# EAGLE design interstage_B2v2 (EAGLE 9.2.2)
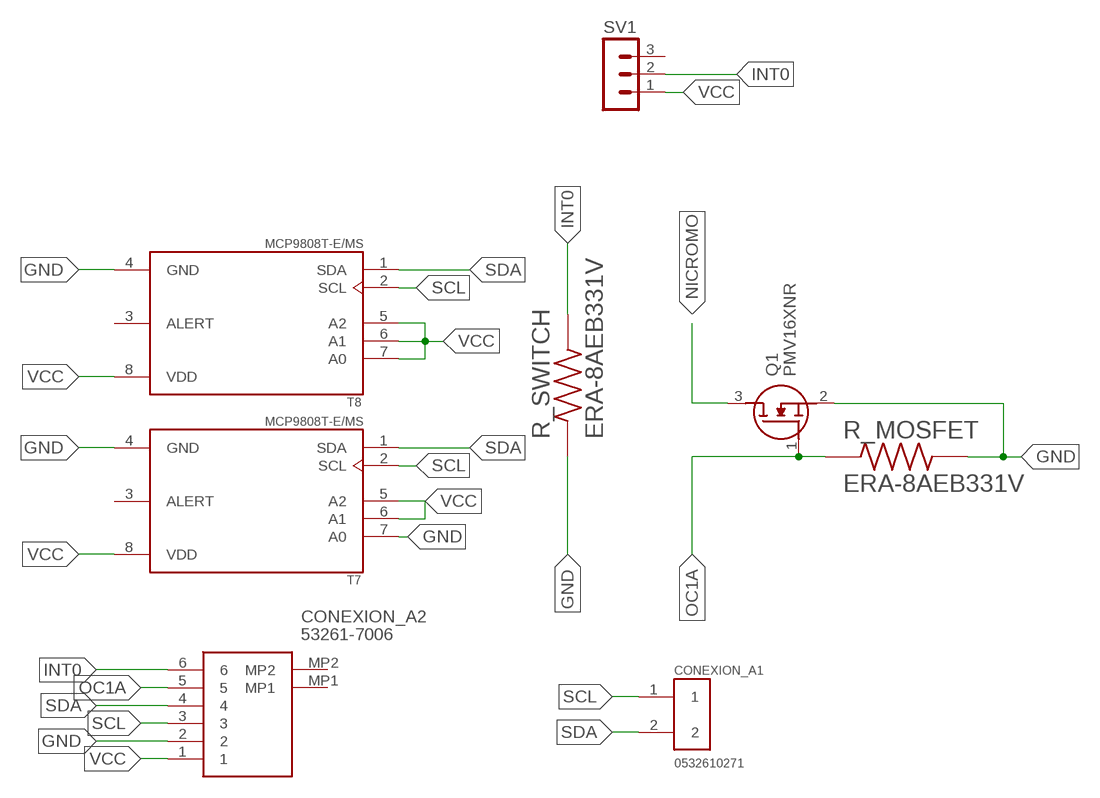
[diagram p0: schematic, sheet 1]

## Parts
CONEXION_A1  0532610271  [MOLEX_0532610271]
CONEXION_A2  53261-7006  [532617006]
Q1  PMV16XNR  [SOT95P230X110-3N]
R_MOSFET  ERA-8AEB331V  [RESC3216X70N]
R_SWITCH  ERA-8AEB331V  [RESC3216X70N]
SV1  MA03-1  [MA03-1]
T7  MCP9808T-E/MS  [SOP65P490X110-8N]
T8  MCP9808T-E/MS  [SOP65P490X110-8N]

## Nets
GND: CONEXION_A2.2 Q1.2(S) R_MOSFET.2 R_SWITCH.1 T7.4(GND) T7.7(A0) T8.4(GND)
INT0: CONEXION_A2.6 R_SWITCH.2 SV1.2
NICROMO: Q1.3(D)
OC1A: CONEXION_A2.5 Q1.1(G) R_MOSFET.1
SCL: CONEXION_A1.1 CONEXION_A2.3 T7.2(SCL) T8.2(SCL)
SDA: CONEXION_A1.2 CONEXION_A2.4 T7.1(SDA) T8.1(SDA)
VCC: CONEXION_A2.1 SV1.1 T7.5(A2) T7.6(A1) T7.8(VDD) T8.5(A2) T8.6(A1) T8.7(A0) T8.8(VDD)
Unconnected: CONEXION_A2.MP1 CONEXION_A2.MP2 SV1.3 T7.3(ALERT) T8.3(ALERT)

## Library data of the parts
CONEXION_A1 = picoblade2:0532610271: 1.25mm (.049") Pitch PicoBlade Header, Surface Mount, Right Angle, Lead-free, 2 Circuits; AVAILABILITY: Unavailable; DESCRIPTION: Picoblade Connector, 2 Circuit Single Row, Right Angle Surface Mount SMT PCB; DIGIKEY-PURCHASE-URL: https://snapeda.com/shop?store=DigiKey&id=4477935; MF: Molex; MP: 0532610271; PACKAGE: None; PRICE: None
CONEXION_A2 = SamacSys_Parts:53261-7006: 1.25mm Pitch, PicoBlade PCB Header, Single Row, Right-Angle, Surface Mount, Gold (Au) Plating, Friction Lock, Circuits, Tape and Reel Source: Datasheet; DESCRIPTION: 1.25mm Pitch, PicoBlade PCB Header, Single Row, Right-Angle, Surface Mount, Gold (Au) Plating, Friction Lock, Circuits, Tape and Reel; HEIGHT: 3.6mm; MANUFACTURER_NAME: Molex; MANUFACTURER_PART_NUMBER: 53261-7006; MOUSER_PART_NUMBER: 538-53261-7006; MOUSER_PRICE-STOCK: https://www.mouser.co.uk/ProductDetail/Molex/53261-7006?qs=0lSvoLzn4L%2FSBef0BTU2GA%3D%3D
Q1 = SamacSys_Parts:PMV16XNR: Nexperia PMV16XNR N-channel MOSFET, 8.6 A, 20 V PMV16XN, 3-Pin SOT-23 Source: Datasheet; DESCRIPTION: Nexperia PMV16XNR N-channel MOSFET, 8.6 A, 20 V PMV16XN, 3-Pin SOT-23; HEIGHT: 1.1mm; MANUFACTURER_NAME: Nexperia; MANUFACTURER_PART_NUMBER: PMV16XNR; MOUSER_PART_NUMBER: 771-PMV16XNR; MOUSER_PRICE-STOCK: https://www.mouser.com/Search/Refine.aspx?Keyword=771-PMV16XNR
R_MOSFET R_SWITCH = resistor_330_smd:ERA-8AEB331V; DESCRIPTION: 330 Ohms ±0.1% 0.25W, 1/4W Chip Resistor 1206 (3216 Metric) Automotive AEC-Q200 Thin Film; DIGI-KEY_PART_NUMBER: P330BCCT-ND; MF: Panasonic Electronic; MP: ERA-8AEB331V; PACKAGE: 3216 Panasonic Electronic Components
SV1 = con-lstb:MA03-1: PIN HEADER; OC_FARNELL: unknown; OC_NEWARK: unknown
T7 T8 = sensorSPEL:MCP9808T-E/MS: Board Mount Temperature Sensors Silicon temp sensor with I2C interface; DESCRIPTION: Temperature Sensor Digital, Local -40°C ~ 125°C 10 b 8-MSOP; DIGI-KEY_PART_NUMBER: MCP9808T-E/MSCT-ND; MF: Microchip; MP: MCP9808T-E/MS; PACKAGE: MSOP-8 Microchip

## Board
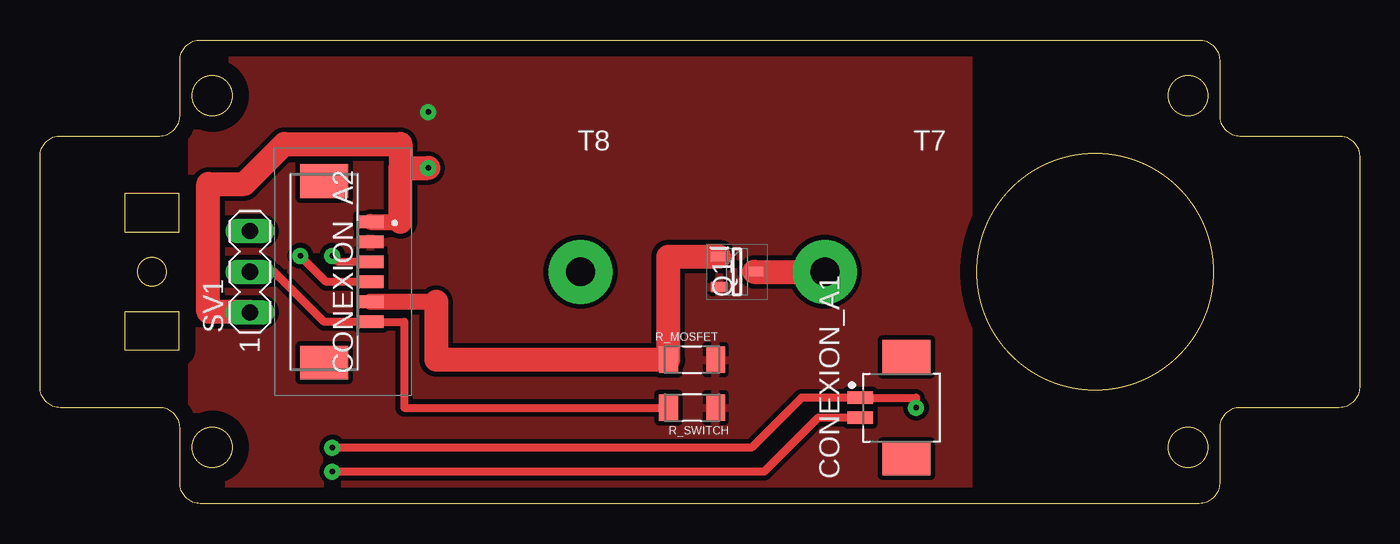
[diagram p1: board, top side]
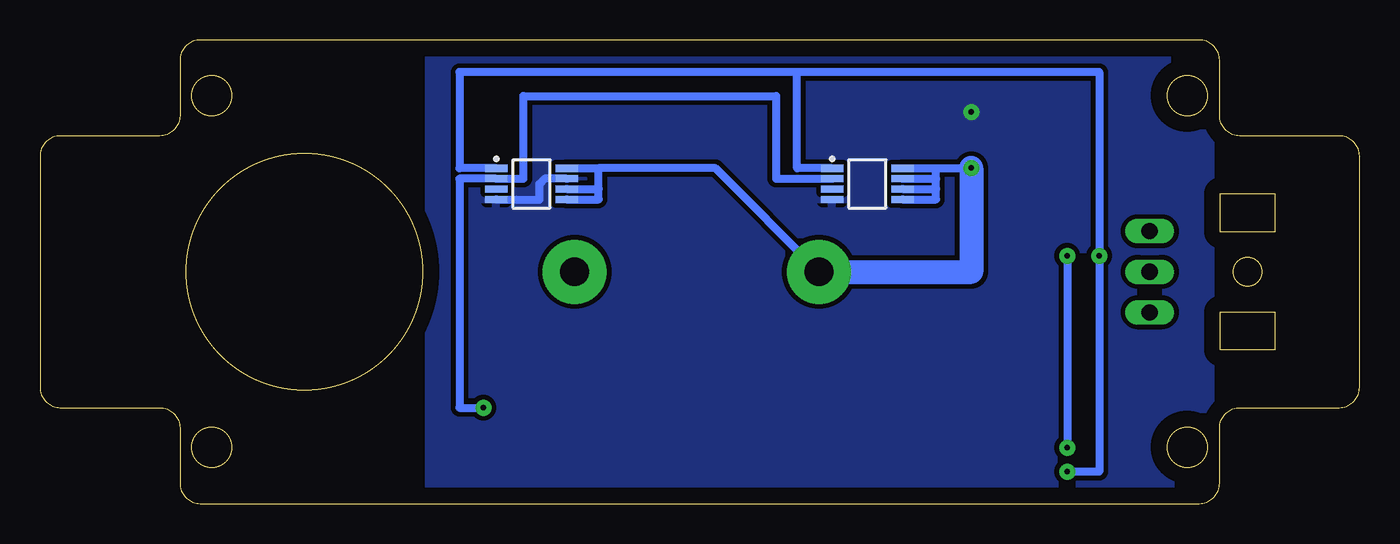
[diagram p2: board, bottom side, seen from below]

Size 82.5 x 29 mm. Coordinates in mm from the lower left corner, seen from the top.
Outline: 8.7,17 8.7,19.4 5.3,19.4 5.3,17 8.7,17
Outline: 8.7,9.6 8.7,12 5.3,12 5.3,9.6 8.7,9.6
Outline: 82.5,21.73 82.5,7.27 arc-90 81.23,6 75.02,6 arc90 73.75,4.73 73.75,1.27 arc-90 72.48,0 10.02,0 arc-90 8.75,1.27 8.75,4.73 arc90 7.48,6 1.27,6 arc-90 0,7.27 0,21.73 arc-90 1.27,23 7.48,23 arc90 8.75,24.27 8.75,27.73 arc-90 10.02,29 72.48,29 arc-90 73.75,27.73 73.75,24.27 arc90 75.02,23 81.23,23 arc-90 82.5,21.73
Outline: circle at 7,14.5 radius 0.9
Outline: circle at 65.97,14.5 radius 7.4
Outline: circle at 71.78,3.52 radius 1.25
Outline: circle at 10.77,25.52 radius 1.25
Outline: circle at 10.77,3.52 radius 1.25
Outline: circle at 71.78,25.52 radius 1.25
Copper layers (1*16): Top 0.035mm / dielectric 1.5mm / Bottom 0.035mm
Design rules "default *": minimum track width 6mil, minimum drill 0.35mm, track to track 0.3mm, track to pad 6mil, pad to pad 6mil, via to via 6mil, smd to smd 6mil, copper to edge 40mil, drill to drill 6mil, minimum pad ring 10mil, minimum via ring 8mil, stop-mask expansion 4mil, vias tented up to drill 0mil, thermal gap 10mil

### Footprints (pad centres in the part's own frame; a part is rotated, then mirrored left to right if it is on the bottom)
MOLEX_0532610271 = smd 0.8 x 1.6: 1 0.625,0; 2 -0.625,0 | smd 2.1 x 3: 3 -3.175,-2.9; 4 3.175,-2.9
532617006 = smd 0.8 x 1.6: 1 3.125,-2.5; 2 1.875,-2.5; 3 0.625,-2.5; 4 -0.625,-2.5; 5 -1.875,-2.5; 6 -3.125,-2.5 | smd 2.1 x 3: MP1 5.675,0.4; MP2 -5.675,0.4
SOT95P230X110-3N = smd 1.05 x 0.6: 1 -1.1,0.95; 2 -1.1,-0.95; 3 1.1,0
RESC3216X70N = smd 1.16 x 1.68: 1 -1.475,0; 2 1.475,0
MA03-1 = drill 1.016 long: 1 -2.54,0; 2 0,0; 3 2.54,0
SOP65P490X110-8N = smd 1.4 x 0.45: 1 -2.2,0.975; 2 -2.2,0.325; 3 -2.2,-0.325; 4 -2.2,-0.975; 5 2.2,-0.975; 6 2.2,-0.325; 7 2.2,0.325; 8 2.2,0.975

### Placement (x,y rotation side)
CONEXION_A1  51.27,6 90 top
CONEXION_A2  18.17,14.5 90 top
Q1  43.57,14.5 0 top
R_MOSFET  40.77,9 0 top
R_SWITCH  40.77,6 180 top
SV1  13.12,14.5 90 top
T7  51.77,20 0 bottom
T8  30.77,20 0 bottom

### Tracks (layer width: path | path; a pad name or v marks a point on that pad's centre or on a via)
GND  (via drill 0.35 pad 1)
  Bottom 0.5: T7.7 50.94,20.32 51.27,20 51.27,19 51.3,19.02 T7.4
  other vias: 24.27,24.5
  pour Top: 9.47,28 9.47,0.6 58.07,0.6 58.07,28.1 57.97,28
  pour Bottom: 9.32,28 9.32,0.4 58.17,0.4 58.17,28
INT0
  Top 0.5: SV1.2 14.64,14.5 17.77,11.38 CONEXION_A2.6 22.77,11.38 22.77,6 R_SWITCH.2
NICROMO  (via drill 1.8 pad 4)
  Top 1.5: Q1.3 v49.07,14.5
OC1A
  Top 0.5: R_MOSFET.1 39.27,9.03
  Top 1: 24.77,12.62 CONEXION_A2.5
  Top 1.5: Q1.1 39.27,15.45 39.27,9.03 | 24.77,12.62 24.77,9 R_MOSFET.1
SCL  (via drill 0.35 pad 1)
  Top 0.5: v54.77,6 54.77,6.62 CONEXION_A1.1 47.59,6.62 44.47,3.5 v18.27,3.5 | CONEXION_A2.3 18.64,15.12 v18.27,15.5
  Bottom 0.5: T8.2 36.47,20.32 36.47,25.5 52.27,25.5 52.27,20.32 T7.2 56.27,20.32 56.27,6 v54.77,6 | v18.27,15.5 v18.27,3.5
SDA  (via drill 0.35 pad 1)
  Top 0.5: CONEXION_A1.2 48.64,5.38 45.27,2 v18.27,2 | CONEXION_A2.4 17.89,13.88 v16.27,15.5
  Bottom 0.5: T8.1 35.17,20.98 35.17,27 | T7.1 56.27,20.98 56.27,27 35.17,27 | 35.17,27 16.27,27 v16.27,15.5 16.27,2 v18.27,2
VCC  (via drill 0.35 pad 1, 1.8 pad 4)
  Top 0.5: SV1.1 13.08,12
  Top 1: CONEXION_A2.1 22.55,17.62
  Top 1.5: 22.55,17.62 22.55,21 | 22.55,21 v24.27,21 | 13.08,12 10.52,12 10.52,20 12.77,20 15.27,22.5 22.55,22.5 22.55,21
  Bottom 0.5: T8.8 26.47,20.98 | T7.8 47.57,20.98 | T8.7 26.47,20.32 | 26.47,20.32 26.47,20.98 | T8.6 26.47,19.68 | 26.47,19.68 26.47,20.32 | T8.5 26.47,19.02 26.47,19.68 | T7.6 47.57,19.68 | 47.57,19.68 47.57,20.98 | T7.5 47.57,19.02 47.57,19.68 | 26.47,20.98 24.27,20.98 v24.27,21 | v33.8,14.5 40.27,20.98 47.57,20.98
  Bottom 1.5: v24.27,21 24.27,14.5 v33.8,14.5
